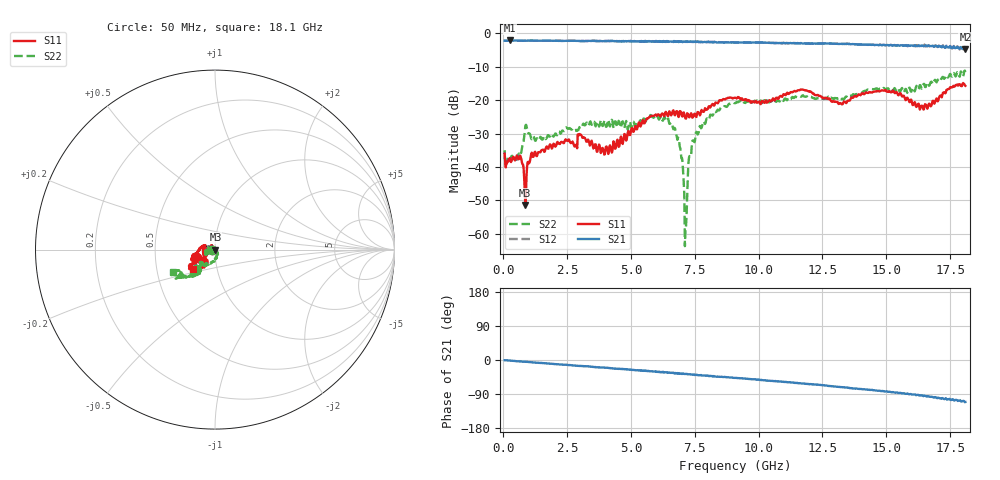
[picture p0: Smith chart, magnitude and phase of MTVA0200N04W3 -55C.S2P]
! Network Analyzer HP8720D.06.14 Serial No. US36140669
! 17 Jan 2005  12:49:50
! Frequency  S11  S21  S12  S22
# HZ  S  DB R 50
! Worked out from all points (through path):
!   801 points, 50 MHz to 18.1 GHz, reference 50 ohm
!   highest |S21| = -2.14 dB at 253.1 MHz (marker M1); lowest = -4.7 dB at 18.1 GHz (marker M2)
!   group delay of S21, straight-line fit = 16 ps
!   lowest |S11| = -51.3 dB at 862.2 MHz (marker M3), VSWR 1.01, Z = 50.3 + j0.0524 ohm
!   |S11| at or under -10 dB: start of sweep to end of sweep
!   |S22| runs from -63.7 to -11.1 dB; largest |S21 - S12| = 0.03
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5e7  -36.04 -167.8  -2.21 -0.6  -2.22 -0.9  -34.99 -178.8
2.530625e8  -37.39 168.8  -2.14 -1.4  -2.16 -1.7  -37.62 -171.8
6.140625e8  -37.59 151.5  -2.19 -3.7  -2.20 -3.8  -36.00 -159.5
8.6225e8  -51.35 11.1  -2.20 -4.7  -2.18 -4.9  -27.63 -151.6
1.178125e9  -36.98 170.9  -2.18 -6.7  -2.21 -6.9  -30.77 164.7
2.802625e9  -33.88 138.9  -2.26 -14.5  -2.23 -15.2  -29.16 150.5
3.073375e9  -30.71 128.9  -2.28 -16.0  -2.24 -16.2  -28.19 -162.9
4.178938e9  -33.53 155.1  -2.28 -21.2  -2.32 -21.5  -27.89 -163.6
6.074188e9  -24.26 -155.5  -2.53 -31.6  -2.52 -31.9  -25.45 -163.3
6.796188e9  -23.29 -157.8  -2.56 -35.0  -2.56 -35.3  -30.94 161.8
6.954125e9  -23.55 -173.8  -2.50 -35.5  -2.52 -35.5  -35.77 140.6
7.066938e9  -23.67 -178.6  -2.43 -36.6  -2.55 -37.1  -44.71 126.7
7.134625e9  -25.48 175.8  -2.49 -37.1  -2.44 -37.3  -59.04 -74.6
7.202312e9  -23.92 175.3  -2.41 -37.1  -2.53 -38.0  -48.39 -13.3
7.337688e9  -24.08 169.0  -2.45 -38.2  -2.48 -38.7  -36.98 -57.8
7.631e9  -23.60 159.8  -2.51 -40.3  -2.56 -40.6  -29.98 -71.6
9.075e9  -19.30 -157.8  -2.74 -47.1  -2.74 -47.5  -20.92 -117.5
1.209838e10  -17.83 -150.6  -3.01 -64.3  -3.05 -64.7  -19.17 -139.3
1.320394e10  -20.90 -145.1  -3.16 -71.1  -3.14 -71.6  -19.96 -133.5
1.509919e10  -17.45 -135.0  -3.67 -84.0  -3.57 -85.0  -16.75 -139.9
1.638525e10  -21.65 -129.0  -3.80 -93.5  -3.74 -95.1  -16.58 -129.2
1.81e10  -15.71 -139.7  -4.66 -110.9  -4.46 -112.5  -11.56 -152.1
